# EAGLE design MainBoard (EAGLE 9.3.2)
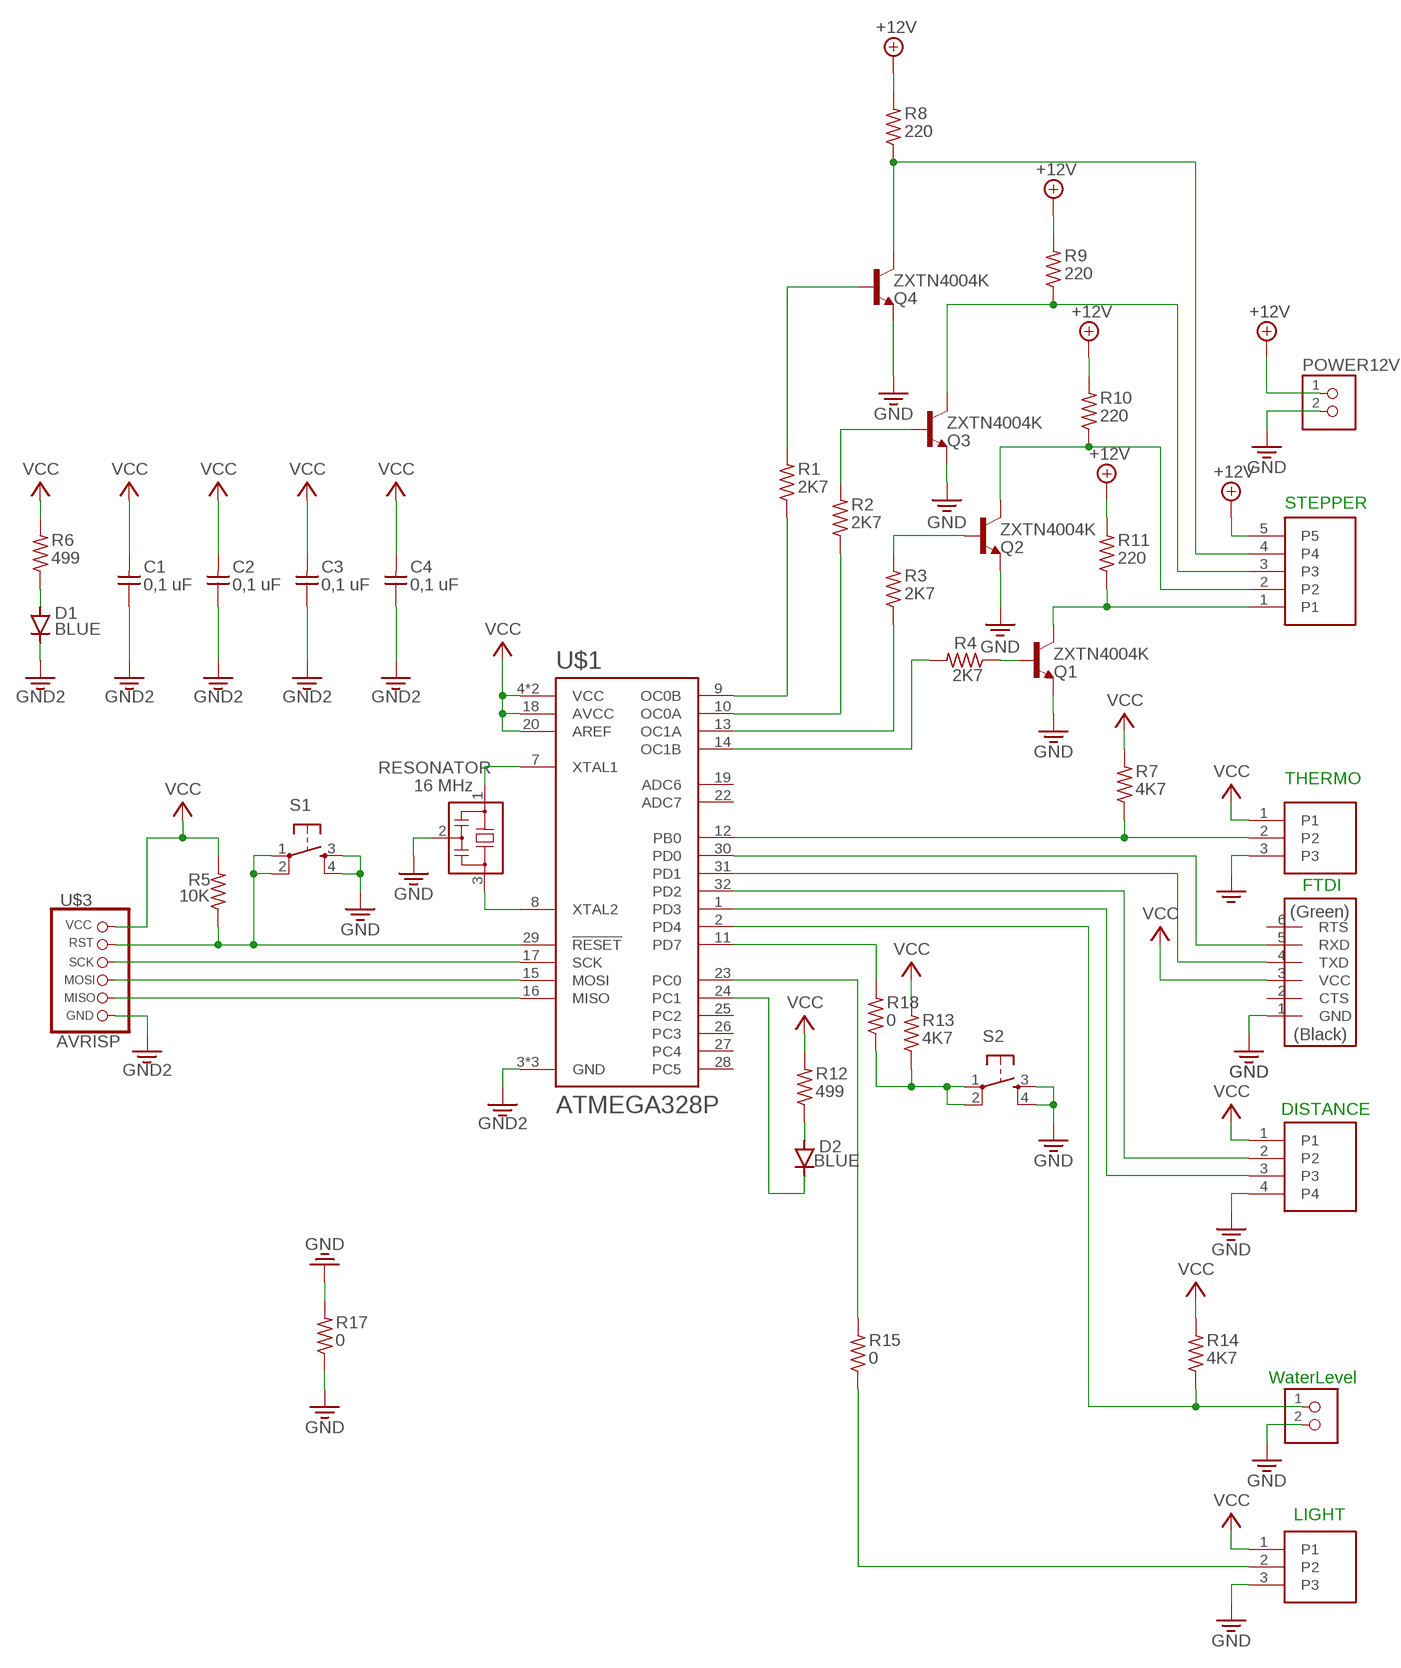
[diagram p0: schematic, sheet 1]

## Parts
C1  0,1 uF  CAP-UNPOLARIZED  [C1206]
C2  0,1 uF  CAP-UNPOLARIZED  [C1206]
C3  0,1 uF  CAP-UNPOLARIZED  [C1206]
C4  0,1 uF  CAP-UNPOLARIZED  [C1206]
D1  BLUE  CDBM1100-G  [MINI-SMA]
D2  BLUE  CDBM1100-G  [MINI-SMA]
LIGHT  LIGHT  HEADERPIN_X3  [1X03SMD]
POWER12V  HEADERPIN_X2  [1X02SMD]
Q1  ZXTN4004K  [TO252]
Q2  ZXTN4004K  [TO252]
Q3  ZXTN4004K  [TO252]
Q4  ZXTN4004K  [TO252]
R1  2K7  RES-US1206  [R1206]
R2  2K7  RES-US1206  [R1206]
R3  2K7  RES-US1206  [R1206]
R4  2K7  RES-US1206  [R1206]
R5  10K  RES-US1206  [R1206]
R6  499  RES-US1206  [R1206]
R7  4K7  RES-US1206  [R1206]
R8  220  RES-US1206  [R1206]
R9  220  RES-US1206  [R1206]
R10  220  RES-US1206  [R1206]
R11  220  RES-US1206  [R1206]
R12  499  RES-US1206  [R1206]
R13  4K7  RES-US1206  [R1206]
R14  4K7  RES-US1206  [R1206]
R15  0  RES-US1206  [R1206]
R17  0  RES-US1206  [R1206]
R18  0  RES-US1206  [R1206]
RESONATOR  16 MHz  RESONATOR  [EFOBM]
S1  6MM_SWITCH6MM_SWITCH  [6MM_SWITCH]
S2  6MM_SWITCH6MM_SWITCH  [6MM_SWITCH]
THERMO  THERMO  HEADERPIN_X3  [1X03SMD]
U$1  ATMEGA328P  ATMEGA328P-AU-2  [QFP80P900X900X120-32N]
U$3  AVRISP  AVRISP_2SMD  [2X03SMD]
U$4  HEADERPIN_X5  [1X05SMD]
U$5  FTDI-SMD-HEADER  [1X06SMD]
U$6  HEADERPIN_X4  [1X04SMD]
U$7  HEADERPIN_X2  [1X02SMD]

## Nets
+12V: POWER12V.1 R8.2 R9.2 R10.2 R11.2 U$4.5
GND: C1.1 C2.1 C3.1 C4.1 D1.KATHODE LIGHT.3 POWER12V.2 Q1.2(E) Q2.2(E) Q3.2(E) Q4.2(E) R17.1 R17.2 RESONATOR.2 S1.3(S) S1.4(S1) S2.3(S) S2.4(S1) THERMO.3 U$1.3(GND) U$1.5(GND) U$1.21(GND) U$3.6(GND) U$5.1(GND) U$6.4 U$7.2 ; supply symbol labelled GND2
N$1: RESONATOR.1 U$1.7(XTAL1)
N$2: RESONATOR.3 U$1.8(XTAL2)
N$3: D1.ANODE R6.1
N$4: U$1.17(SCK) U$3.3(SCK)
N$5: U$1.15(MOSI) U$3.4(MOSI)
N$6: U$1.16(MISO) U$3.1(MISO)
N$7: R4.2 U$1.14(OC1B)
N$8: R3.1 U$1.13(OC1A)
N$9: R2.1 U$1.10(OC0A)
N$10: Q4.1(B) R1.2
N$11: Q1.3(C) R11.1 U$4.1
N$12: Q2.3(C) R10.1 U$4.2
N$13: Q3.3(C) R9.1 U$4.3
N$14: Q4.3(C) R8.1 U$4.4
N$15: Q1.1(B) R4.1
N$16: Q2.1(B) R3.2
N$17: Q3.1(B) R2.2
N$18: R1.1 U$1.9(OC0B)
N$19: R5.1 S1.1(P) S1.2(P1) U$1.29(!RESET) U$3.5(RST)
N$20: R7.1 THERMO.2 U$1.12(PB0)
N$21: D2.ANODE R12.1
N$22: R13.1 R18.1 S2.1(P) S2.2(P1)
N$23: D2.KATHODE U$1.24(PC1)
N$24: R14.1 U$1.2(PD4) U$7.1
N$26: U$1.32(PD2) U$6.2
N$27: U$1.1(PD3) U$6.3
N$28: U$1.31(PD1) U$5.4(TXD)
N$29: U$1.30(PD0) U$5.5(RXD)
N$30: R15.2 U$1.23(PC0)
N$31: R18.2 U$1.11(PD7)
N$32: LIGHT.2 R15.1
VCC: C1.2 C2.2 C3.2 C4.2 LIGHT.1 R5.2 R6.2 R7.2 R12.2 R13.2 R14.2 THERMO.1 U$1.4(VCC) U$1.6(VCC) U$1.18(AVCC) U$1.20(AREF) U$3.2(VCC) U$5.3(VCC) U$6.1
Unconnected: U$1.19(ADC6) U$1.22(ADC7) U$1.25(PC2) U$1.26(PC3) U$1.27(PC4) U$1.28(PC5) U$5.2(CTS) U$5.6(RTS)

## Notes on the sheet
- STEPPER
- THERMO
- FTDI
- DISTANCE
- WaterLevel
- LIGHT

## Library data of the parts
C1-C4 = Fablab:CAP-UNPOLARIZED
D1 D2 = Fablab:CDBM1100-G: Diode schottky 100V 1A mini-SMA as found in the fablab inventory
LIGHT THERMO = Fablab:HEADERPIN_X3
POWER12V U$7 = Fablab:HEADERPIN_X2
Q1-Q4 = Fablab:ZXTN4004K: NPN Transistor
R1-R15 R17 R18 = Fablab:RES-US: Resistor (US Symbol)
RESONATOR = Fablab:RESONATOR
S1 S2 = Fablab:6MM_SWITCH: OMRON SWITCH
U$1 = ATMEGA328P-AU:ATMEGA328P-AU-2
U$3 = Fablab:AVRISP_2
U$4 = Fablab:HEADERPIN_X5
U$5 = Fablab:FTDI-SMD-HEADER
U$6 = Fablab:HEADERPIN_X4

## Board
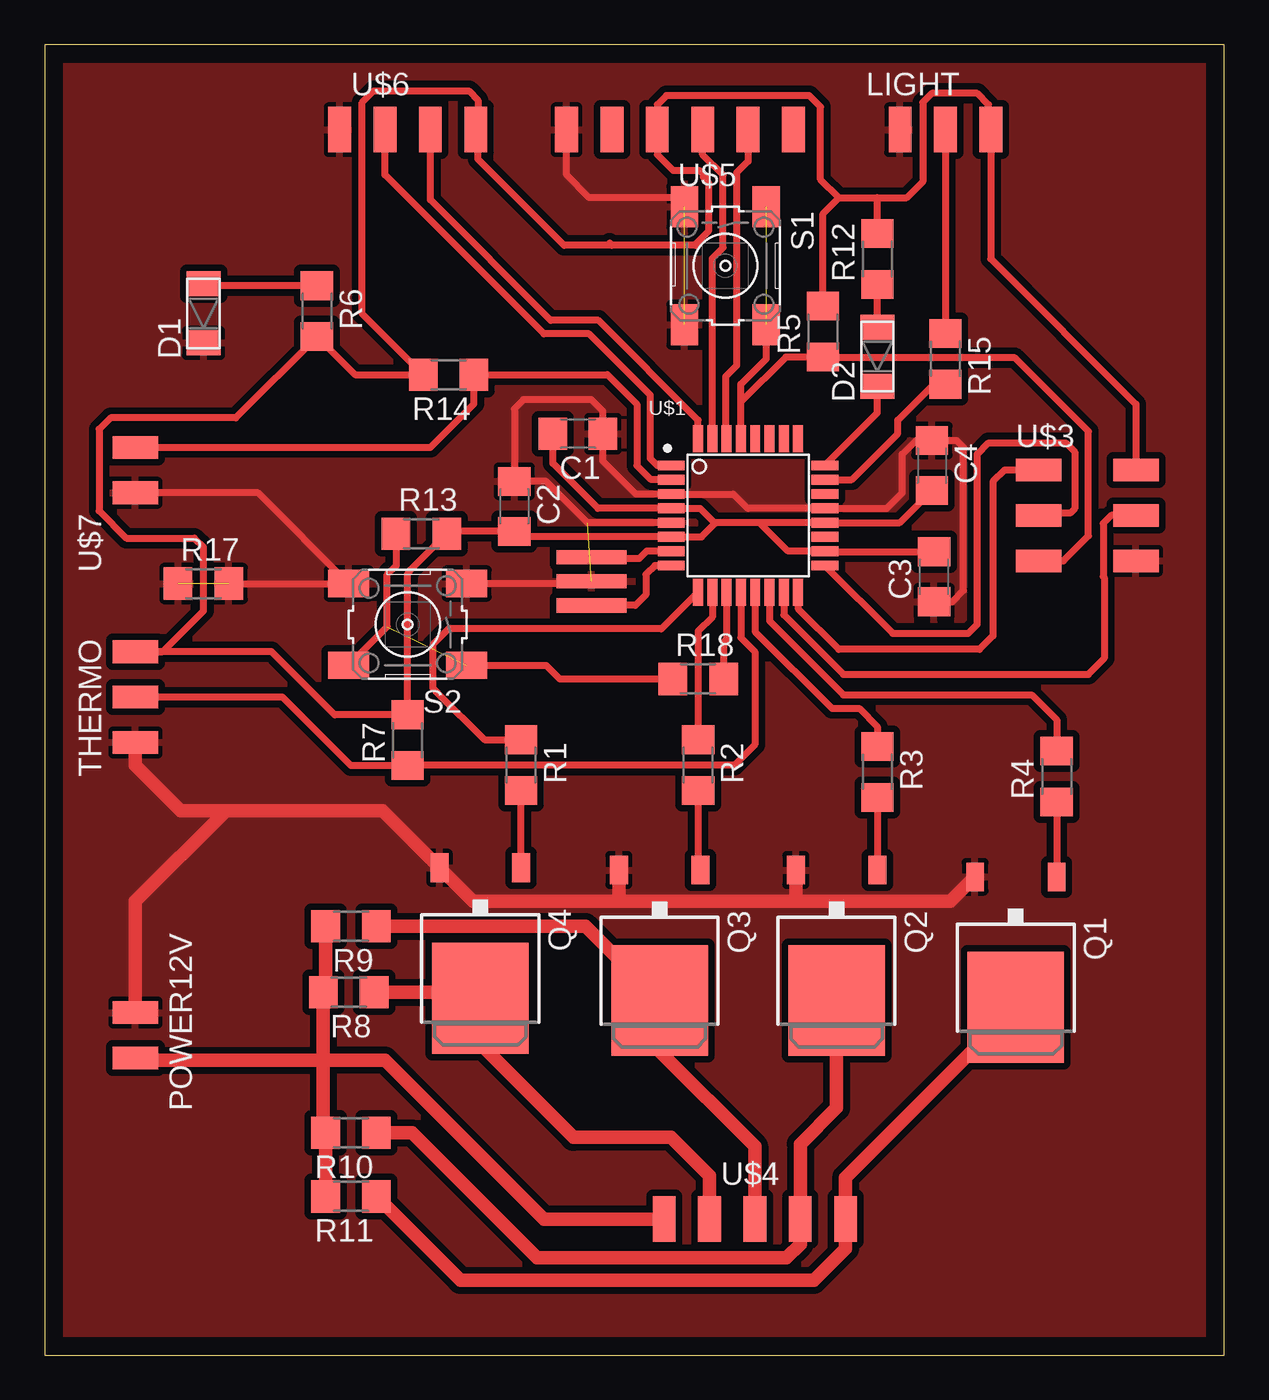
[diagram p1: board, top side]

Size 66.02 x 73.33 mm. Coordinates in mm from the lower left corner, seen from the top.
Outline: 0,0 66.02,0 66.02,73.33 0,73.33 0,0
Copper layers (1*16): Top 0.035mm / dielectric 1.5mm / Bottom 0.035mm
Design rules "default *": minimum track width 6mil, minimum drill 0.35mm, track to track 15mil, track to pad 15mil, pad to pad 15mil, via to via 5mil, smd to smd 6mil, copper to edge 40mil, drill to drill 6mil, minimum pad ring 10mil, minimum via ring 8mil, stop-mask expansion 4mil, vias tented up to drill 0mil, thermal gap 10mil

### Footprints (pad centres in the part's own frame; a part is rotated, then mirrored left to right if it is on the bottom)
C1206 = smd 1.6 x 1.8: 1 -1.4,0; 2 1.4,0
MINI-SMA = smd 1.4 x 1.9: ANODE 1.65,0; KATHODE -1.65,0
1X03SMD = smd 2.54 x 1.27: 1 0,3.81; 2 0,1.27; 3 0,-1.27
1X02SMD = smd 2.54 x 1.27: 1 0,3.81; 2 0,1.27
TO252 = smd 1 x 1.6: 1 -2.28,-6.07; 2 2.28,-6.07 | smd 5.4 x 6.2: 3 0,1.23
R1206 = smd 1.6 x 1.803: 1 -1.422,0; 2 1.422,0
EFOBM = smd 0.8 x 3.9: 1 -1.35,0; 2 0,0; 3 1.35,0
6MM_SWITCH = smd 2.286 x 1.524: 1 -3.302,2.286; 2 3.302,2.286; 3 -3.302,-2.286; 4 3.302,-2.286
QFP80P900X900X120-32N = smd 1.5 x 0.55: 1 -4.3,2.8; 2 -4.3,2; 3 -4.3,1.2; 4 -4.3,0.4; 5 -4.3,-0.4; 6 -4.3,-1.2; 7 -4.3,-2; 8 -4.3,-2.8; 17 4.3,-2.8; 18 4.3,-2; 19 4.3,-1.2; 20 4.3,-0.4; 21 4.3,0.4; 22 4.3,1.2; 23 4.3,2; 24 4.3,2.8 | smd 0.55 x 1.5: 9 -2.8,-4.3; 10 -2,-4.3; 11 -1.2,-4.3; 12 -0.4,-4.3; 13 0.4,-4.3; 14 1.2,-4.3; 15 2,-4.3; 16 2.8,-4.3; 25 2.8,4.3; 26 2,4.3; 27 1.2,4.3; 28 0.4,4.3; 29 -0.4,4.3; 30 -1.2,4.3; 31 -2,4.3; 32 -2.8,4.3
2X03SMD = smd 2.54 x 1.27: 1 -2.54,2.54; 2 2.92,2.54; 3 -2.54,0; 4 2.92,0; 5 -2.54,-2.54; 6 2.92,-2.54
1X05SMD = smd 2.54 x 1.27: 1 0,3.81; 2 0,1.27; 3 0,-1.27; 4 0,-3.81; 5 0,-6.35
1X06SMD = smd 2.54 x 1.27: 1 0,6.35; 2 0,3.81; 3 0,1.27; 4 0,-1.27; 5 0,-3.81; 6 0,-6.35
1X04SMD = smd 2.54 x 1.27: 1 0,3.81; 2 0,1.27; 3 0,-1.27; 4 0,-3.81

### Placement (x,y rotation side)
C1  29.85,51.56 180 top
C2  26.29,47.5 270 top
C3  49.78,43.56 90 top
C4  49.66,49.78 270 top
D1  8.89,58.29 90 top
D2  46.61,55.88 90 top
LIGHT  49.15,68.58 270 top
POWER12V  5.08,20.45 180 top
Q1  54.36,20.7 180 top
Q2  44.32,21.08 180 top
Q3  34.42,21.08 180 top
Q4  24.38,21.21 180 top
R1  26.67,33.02 270 top
R2  36.58,33.02 270 top
R3  46.61,32.64 270 top
R4  56.64,32.39 90 top
R5  43.56,57.28 90 top
R6  15.24,58.42 270 top
R7  20.32,34.42 90 top
R8  17.02,20.32 180 top
R9  17.14,24 180 top
R10  17.14,12.45 180 top
R11  17.14,8.89 180 top
R12  46.61,61.34 90 top
R13  21.08,45.97 0 top
R14  22.61,54.86 180 top
R15  50.42,55.75 270 top
R17  8.89,43.18 0 top
R18  36.58,37.85 0 top
RESONATOR  30.61,43.31 270 top
S1  38.1,60.96 270 top
S2  20.32,40.89 180 top
THERMO  5.08,35.56 0 top
U$1  39.37,46.99 0 top
U$3  58.17,46.99 0 top
U$4  41.02,7.62 270 top
U$5  35.56,68.58 90 top
U$6  20.32,68.58 270 top
U$7  5.08,46.99 0 top

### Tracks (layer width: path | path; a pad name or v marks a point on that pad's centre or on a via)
+12V
  Top 0.762: R9.2 15.72,20.45 R8.2 15.6,16.51 | 15.6,16.51 15.6,12.57 R10.2 R11.2 | 15.6,16.51 19.05,16.51 27.94,7.62 U$4.5 | POWER12V.1 5.21,16.51 15.6,16.51
GND  (3 unrouted)
  Top 0.381: U$1.5 30.37,46.59 28.06,48.9 C2.1 26.29,52.96 26.8,53.47 30.61,53.47 31.25,52.83 C1.1 31.25,50.04 33.09,48.19 U$1.3 38.55,48.19 39.37,47.37 39.39,47.39 U$1.21 47.14,47.39 48.01,48.26 48.01,50.42 48.77,51.18 C4.1 51.05,51.18 51.44,50.8 51.44,42.8 50.8,42.16 C3.1 | RESONATOR.2 30.48,43.18 S2.3 | U$7.2 11.94,48.26 S2.4 R17.2 | S1.3 35.31,64.77 30.48,64.77 29.21,66.04 U$5.1
  Top 0.762: Q1.2 50.7,25.4 42.04,25.4 | 42.04,25.4 32.13,25.4 | 32.13,25.4 23.98,25.4 Q4.2 18.9,30.48 10.16,30.48 | Q3.2 32.14,25.41 32.13,25.4 | Q2.2 42.04,25.41 42.04,25.4 | 10.16,30.48 7.62,30.48 5.08,33.02 THERMO.3 | POWER12V.2 5.08,25.4 10.16,30.48
  pour Top: 0,0 0,73.41 66.04,73.41 66.04,0
N$1
  Top 0.381: U$1.7 33.69,44.99 33.27,44.58 30.69,44.58 RESONATOR.1
N$2
  Top 0.381: U$1.8 34.16,44.19 33.66,43.69 33.66,42.55 33.07,41.96 RESONATOR.3
N$3
  Top 0.381: R6.1 8.99,59.84 D1.ANODE
N$4
  Top 0.381: U$1.17 47.47,40.39 51.69,40.39 52.2,40.89 52.2,50.42 52.83,51.05 57.15,51.05 57.66,50.55 57.66,47.37 57.4,47.12 55.75,47.12 U$3.3
N$5
  Top 0.381: U$3.4 59.69,46.99 59.24,46.54 59.24,43.58 59.31,43.51 59.31,38.99 58.42,38.1 44.7,38.1 41.37,41.43 U$1.15
N$6
  Top 0.381: U$3.1 53.72,49.53 53.09,48.9 53.09,40.26 52.32,39.5 44.45,39.5 42.17,41.78 U$1.16
N$7
  Top 0.381: U$1.14 40.57,41.09 44.7,36.96 55.25,36.96 56.64,35.56 R4.2
N$8
  Top 0.381: U$1.13 39.77,40.49 44.07,36.2 45.59,36.2 46.61,35.18 R3.1
N$9
  Top 0.381: U$1.10 37.37,41.31 36.58,40.51 R2.1
N$10
  Top 0.381: Q4.1 R1.2
N$11
  Top 0.762: Q1.3 44.83,9.95 U$4.1 44.83,5.97 43.05,4.19 23.27,4.19 R11.1
N$12
  Top 0.762: R10.1 20.57,12.45 27.56,5.46 41.53,5.46 42.29,6.22 U$4.2 42.29,11.81 44.32,13.84 Q2.3
N$13
  Top 0.762: R9.1 30.27,24 Q3.3 34.42,17.02 39.75,11.68 U$4.3
N$14
  Top 0.762: R8.1 24.04,20.32 Q4.3 24.38,17.4 29.59,12.19 35.05,12.19 37.21,10.03 U$4.4
N$15
  Top 0.381: R4.1 Q1.1
N$16
  Top 0.381: R3.2 Q2.1
N$17
  Top 0.381: R2.2 36.58,27.27 Q3.1
N$18
  Top 0.381: U$1.9 34.52,40.64 22.61,40.64 21.72,39.75 21.72,37.34 21.91,37.15 21.97,37.08 24.61,34.44 R1.1
N$19  (1 unrouted)
  Top 0.381: U$3.5 57.02,44.45 58.42,45.85 58.42,51.69 54.31,55.8 43.61,55.8 R5.1 41.48,55.86 38.97,53.34 | U$1.29 38.97,53.34 | 38.97,53.34 38.97,54.34 40.39,55.75 S1.2
N$20
  Top 0.381: U$1.12 38.97,40.15 39.75,39.37 39.75,34.16 38.61,33.02 20.34,33.02 R7.1 17.14,33 13.31,36.83 THERMO.2
N$21
  Top 0.381: D2.ANODE R12.1
N$22  (1 unrouted)
  Top 0.381: S2.2 19.18,40.77 19.18,43.69 19.68,44.2 19.68,45.95 R13.1 | S2.1 28.07,38.61 28.83,37.85 R18.1
N$23
  Top 0.381: U$1.24 46.61,52.73 D2.KATHODE
N$24
  Top 0.381: U$1.2 33.94,48.99 33.15,49.78 33.15,53.21 31.5,54.86 R14.1 24.03,53.24 21.59,50.8 U$7.1
N$26
  Top 0.381: U$1.32 36.57,52.33 30.99,57.91 28.32,57.91 21.59,64.64 U$6.2
N$27
  Top 0.381: U$1.1 34.28,49.79 33.91,50.16 33.91,53.72 30.48,57.15 27.94,57.15 19.05,66.04 U$6.3
N$28
  Top 0.381: U$1.31 37.37,61.37 37.97,61.98 37.97,66.04 36.83,67.18 U$5.4
N$29
  Top 0.381: U$5.5 39.37,66.8 38.73,66.17 38.73,55.37 38.13,54.77 38.13,54.74 38.13,51.33 U$1.30
N$30
  Top 0.381: U$1.23 45.18,48.99 47.75,51.56 47.75,52.32 49.76,54.33 R15.2
N$31
  Top 0.381: U$1.11 38.17,40.08 38,39.9 R18.2
N$32
  Top 0.381: LIGHT.2 R15.1
VCC
  Top 0.381: C1.2 28.45,49.91 30.97,47.39 U$1.4 36.68,47.39 37.53,46.55 | 37.53,46.55 36.77,45.79 U$1.6 26.6,45.79 C2.2 22.63,46.1 R13.2 20.45,43.92 20.45,43.88 20.32,43.75 R7.2 16.23,35.84 12.7,39.37 THERMO.1 6.6,39.37 8.89,41.66 8.89,45.21 8.38,45.72 4.57,45.72 3.05,47.24 3.05,51.82 3.68,52.45 10.69,52.45 R6.2 17.37,54.86 R14.2 17.78,58.27 17.78,70.1 18.41,70.74 23.75,70.74 24.26,70.23 24.26,68.45 | 40,46.59 U$1.20 47.86,46.59 C4.2 | 40,46.59 37.57,46.59 37.53,46.55 | 40,46.59 41.61,44.99 U$1.18 43.7,44.96 C3.2 | 36.86,66.07 36.64,66.29 35.18,66.29 34.29,67.18 U$5.3 34.29,69.98 34.8,70.48 42.8,70.48 43.43,69.85 43.43,65.79 44.45,64.77 | 36.86,66.07 37.08,65.85 | 36.86,66.07 36.86,65.93 37.15,65.64 37.15,62.88 36.45,62.18 36.45,62.1 31.75,62.1 | 31.75,62.1 31.62,62.23 | R5.2 43.56,63.88 44.45,64.77 | 44.45,64.77 46.61,64.77 | 46.61,64.77 48.26,64.77 49.15,65.66 49.15,70.1 49.66,70.61 52.2,70.61 52.83,69.98 52.83,68.71 LIGHT.1 52.96,61.34 61.09,53.21 U$3.2 | R12.2 46.61,64.77 | 24.26,68.45 24.26,66.93 29.08,62.1 31.75,62.1 | 24.26,68.45 U$6.1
